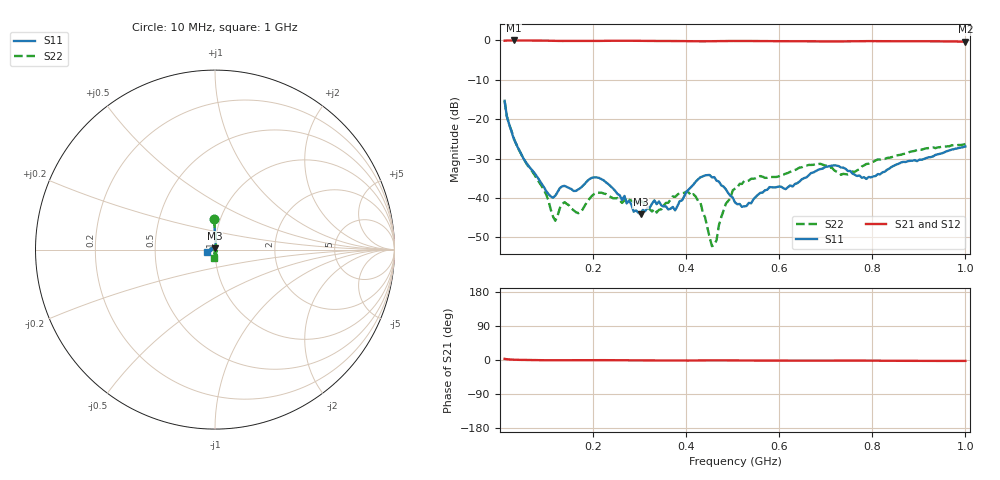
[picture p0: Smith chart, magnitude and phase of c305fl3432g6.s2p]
!Agilent Technologies,N5234A,MY52241123,A.10.00.00
!Agilent N5234A: A.10.00.00
!Date: Wednesday, September 04, 2019 09:47:00
!Correction: S11(Full 2 Port(1,2))
!S21(Full 2 Port(1,2))
!S12(Full 2 Port(1,2))
!S22(Full 2 Port(1,2))
!S2P File: Measurements: S11, S21, S12, S22:
# Hz S  dB  R 50
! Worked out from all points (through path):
!   201 points, 10 MHz to 1 GHz, reference 50 ohm
!   highest |S21| = -0.07 dB at 29.8 MHz (marker M1); lowest = -0.4 dB at 1 GHz (marker M2)
!   lowest |S11| = -44.1 dB at 302.1 MHz (marker M3), VSWR 1.01, Z = 49.9 + j0.614 ohm
!   |S11| at or under -10 dB: start of sweep to end of sweep
!   |S22| runs from -52.2 to -15.4 dB; largest |S21 - S12| = 0.0058
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1e7  -15.36 91.2  -0.13 3.1  -0.11 3.4  -15.41 92.1
2.98e7  -25.02 86.4  -0.07 0.8  -0.06 0.8  -24.84 86.1
9.415e7  -37.21 83.8  -0.10 -0.6  -0.11 -0.5  -37.90 67.6
1.189e8  -39.42 114.6  -0.17 -0.8  -0.17 -0.8  -45.77 99.6
1.387e8  -36.93 113.5  -0.19 -0.6  -0.20 -0.5  -41.06 107.2
1.783e8  -36.86 119.5  -0.21 -0.6  -0.21 -0.6  -42.79 110.5
2.1295e8  -34.91 97.1  -0.18 -0.3  -0.18 -0.3  -38.67 81.3
3.0205e8  -44.13 98.0  -0.16 -1.2  -0.16 -1.1  -40.76 -24.5
3.4165e8  -40.89 124.8  -0.20 -1.2  -0.21 -1.2  -42.99 -40.3
3.763e8  -43.13 150.2  -0.21 -1.4  -0.21 -1.4  -39.73 -60.0
4.159e8  -36.59 153.8  -0.27 -1.4  -0.27 -1.4  -39.07 -97.7
4.3075e8  -34.76 144.1  -0.29 -1.2  -0.30 -1.1  -41.13 -109.8
4.555e8  -34.76 122.8  -0.27 -0.9  -0.26 -0.9  -52.22 -93.6
4.654e8  -35.62 119.3  -0.24 -0.9  -0.24 -0.9  -50.67 -53.2
4.852e8  -37.77 119.2  -0.21 -1.0  -0.21 -1.0  -41.49 -36.2
5.05e8  -41.11 125.9  -0.20 -1.2  -0.20 -1.1  -37.64 -43.6
5.2975e8  -42.04 150.8  -0.20 -1.4  -0.20 -1.4  -35.78 -52.8
6.733e8  -33.55 -173.5  -0.28 -2.0  -0.29 -1.9  -31.60 -84.5
7.4755e8  -33.17 165.7  -0.28 -1.4  -0.29 -1.4  -34.06 -90.2
7.8715e8  -35.17 -175.2  -0.24 -1.6  -0.24 -1.6  -31.39 -73.8
8.3665e8  -32.54 -165.7  -0.25 -2.1  -0.26 -2.1  -29.79 -76.9
1e9  -26.93 -162.5  -0.37 -2.4  -0.37 -2.4  -26.32 -95.4
